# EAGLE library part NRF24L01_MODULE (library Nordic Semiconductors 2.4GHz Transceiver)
This module based on Nordic nRF24L01, highly integrated, ultra low power (ULP) 2Mbps RF transceiver for the 2.4GHz ISM (Industrial, Scientific and Medical) band. Nordic nRF24L01+ integrates a complete 2.4GHz RF transceiver, RF synthesizer, and baseband logic including the Enhanced ShockBurst™ hardware protocol accelerator supporting a high-speed SPI interface for the application controller.
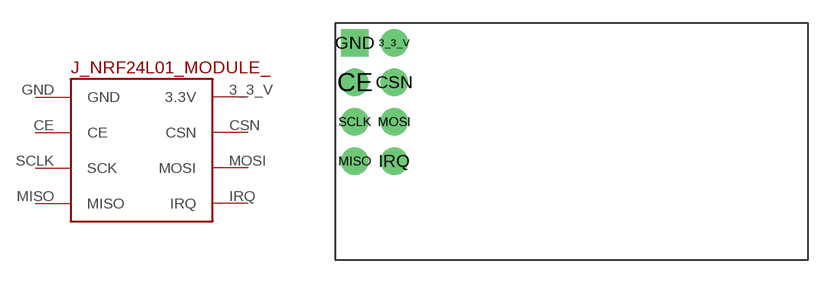
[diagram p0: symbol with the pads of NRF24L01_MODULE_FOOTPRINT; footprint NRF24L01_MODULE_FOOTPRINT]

Designator prefix J_NRF24L01_MODULE_

## NRF24L01_MODULE  [NRF24L01_MODULE_FOOTPRINT]
3_3_V  3.3V
CE  CE
CSN  CSN
GND  GND
IRQ  IRQ
MISO  MISO
MOSI  MOSI
SCLK  SCK

## Footprint NRF24L01_MODULE_FOOTPRINT (pad centres in mm)
This module based on Nordic nRF24L01, highly integrated, ultra low power (ULP) 2Mbps RF transceiver for the 2.4GHz ISM (Industrial, Scientific and Medical) band. Nordic nRF24L01+ integrates a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
drill 0.9 pad 1.778: 3_3_V -11.43,6.35; CE -13.97,3.81; CSN -11.43,3.81; IRQ -11.43,-1.27; MISO -13.97,-1.27; MOSI -11.43,1.27; SCLK -13.97,1.27
drill 0.9 pad 1.778 square: GND -13.97,6.35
